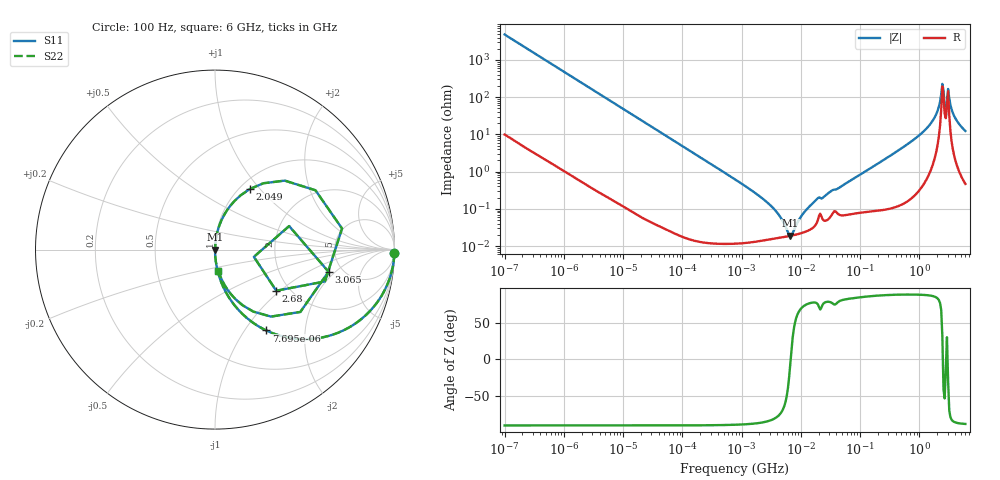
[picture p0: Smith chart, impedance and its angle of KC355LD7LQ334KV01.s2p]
!Murata Part Number: KC355LD7LQ334KV01
!These Parameters are Measured in Series Mode Connection
!Data Generated on Mar 13, 2026
!  o--ll--o
!Port1  Port2
!  o------o
!Operation Temp=25[degC], DC Bias Voltage=0[V]
!Freq. Start=100[Hz] Stop=6[GHz] 401[Steps]
# Hz S RI R 50
!Freq.(Hz) S11(Real) S11(Imag) S21(Real) S21(Imag) S12(Real) S12(Imag) S22(Real) S22(Imag)
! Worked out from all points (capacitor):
!   401 points, 100 Hz to 6 GHz, reference 50 ohm
!   read as one part in series: C = 329 nF near 109 Hz
!   lowest |Z| = 18.9 mohm at 6.644 MHz (marker M1)
!   series resonance near 6.735 MHz, so ESL is about 1.7 nH
!   S11 on the Smith chart (normalised r, x): 100 Hz: 1, -97; 7.695 kHz: 1.00, -1.26; 2.049 GHz: 1.11, +0.88; 2.68 GHz: 1.71, -0.94; 3.065 GHz: 3.89, -1.64; 6 GHz: 1.01, -0.25
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100  0.9995 -0.0207  0.000471 0.0207  0.000471 0.0207  0.9995 -0.0207
548  0.9871 -0.1118  0.0129 0.1118  0.0129 0.1118  0.9871 -0.1118
2008  0.8531 -0.353  0.1469 0.353  0.1469 0.353  0.8531 -0.353
4111  0.5821 -0.4921  0.4179 0.4921  0.4179 0.4921  0.5821 -0.4921
7695  0.2855 -0.4505  0.7145 0.4505  0.7145 0.4505  0.2855 -0.4505
15752  0.0876 -0.2815  0.9124 0.2815  0.9124 0.2815  0.0876 -0.2815
40335  0.0147 -0.1189  0.9853 0.1189  0.9853 0.1189  0.0147 -0.1189
774597  0.000154 -0.0062  0.9998 0.0062  0.9998 0.0062  0.000154 -0.0062
3245845  0.000156 -0.00113  0.9998 0.00113  0.9998 0.00113  0.000156 -0.00113
6644369  0.000188 -1.88e-05  0.9998 1.88e-05  0.9998 1.88e-05  0.000188 -1.88e-05
1.039699e7  0.000225 0.00063  0.9998 -0.00063  0.9998 -0.00063  0.000225 0.00063
1.555665e7  0.000302 0.00134  0.9997 -0.00134  0.9997 -0.00134  0.000302 0.00134
3.124326e8  0.00167 0.0257  0.9983 -0.0257  0.9983 -0.0257  0.00167 0.0257
1.144649e9  0.017 0.1123  0.983 -0.1123  0.983 -0.1123  0.017 0.1123
1.712697e9  0.0697 0.223  0.9303 -0.223  0.9303 -0.223  0.0697 0.223
2.048624e9  0.1931 0.3368  0.8069 -0.3368  0.8069 -0.3368  0.1931 0.3368
2.34314e9  0.5598 0.3305  0.4402 -0.3305  0.4402 -0.3305  0.5598 0.3305
2.679998e9  0.3413 -0.2292  0.6587 0.2292  0.6587 0.2292  0.3413 -0.2292
3.065283e9  0.6326 -0.1233  0.3674 0.1233  0.3674 0.1233  0.6326 -0.1233
3.505958e9  0.2132 -0.3452  0.7868 0.3452  0.7868 0.3452  0.2132 -0.3452
4.193612e9  0.0716 -0.2259  0.9284 0.2259  0.9284 0.2259  0.0716 -0.2259
6e9  0.0194 -0.1203  0.9806 0.1203  0.9806 0.1203  0.0194 -0.1203
